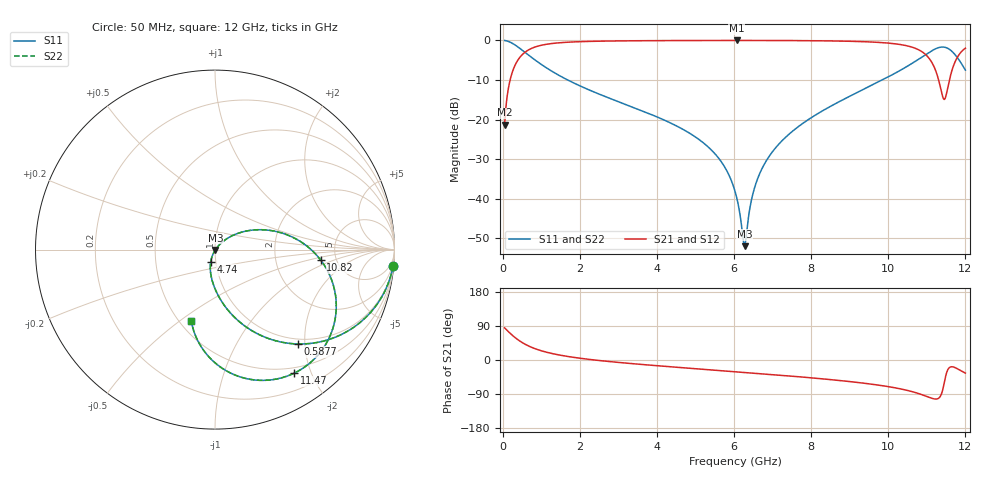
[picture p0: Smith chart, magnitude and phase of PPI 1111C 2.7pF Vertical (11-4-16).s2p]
# GHz S MA R 50
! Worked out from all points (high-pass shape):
!   1601 points, 50 MHz to 12 GHz, reference 50 ohm
!   highest |S21| = -0.02 dB at 6.07 GHz (marker M1); lowest = -21.3 dB at 50 MHz (marker M2)
!   |S21| within 3 dB of the highest: 575.9 MHz to 10.9 GHz (10.32 GHz wide, 180 % of centre); 11.88 GHz to end of sweep
!   lowest |S11| = -52.0 dB at 6.271 GHz (marker M3), VSWR 1.01, Z = 50.2 - j0.133 ohm
!   |S11| at or under -10 dB: 1.683 GHz to 9.847 GHz (8.163 GHz wide, 142 % of centre)
!   |S22| runs from -52.0 to 0.0 dB; largest |S21 - S12| = 0
!   S11 on the Smith chart (normalised r, x): 50 MHz: 1, -22; 587.8 MHz: 0.90, -1.86; 4.74 GHz: 0.94, -0.13; 10.82 GHz: 3.77, -0.68; 11.47 GHz: 0.42, -1.75; 12 GHz: 0.57, -0.55
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0.05  0.9963 -5.2  0.08604 84.8  0.08604 84.8  0.9963 -5.2
0.1545625  0.9661 -15.8  0.258 74.2  0.258 74.2  0.9661 -15.8
0.2516563  0.9169 -24.9  0.3988 65.1  0.3988 65.1  0.9169 -24.9
0.58775  0.7003 -48.7  0.7132 41.3  0.7132 41.3  0.7003 -48.7
1.140437  0.4477 -69.4  0.8932 20.5  0.8932 20.5  0.4477 -69.4
2.044156  0.2606 -85.6  0.9641 4.1  0.9641 4.1  0.2606 -85.6
4.038312  0.106 -104.4  0.9924 -15.4  0.9924 -15.4  0.106 -104.4
4.740375  0.0721 -109.4  0.9952 -20.9  0.9952 -20.9  0.0721 -109.4
5.569406  0.03391 -113.5  0.9969 -27.3  0.9969 -27.3  0.03391 -113.5
6.025  0.01241 -109.7  0.9972 -30.8  0.9972 -30.8  0.01241 -109.7
6.069813  0.01027 -107.5  0.9972 -31.1  0.9972 -31.1  0.01027 -107.5
6.271469  0.002511 -31.8  0.9971 -32.7  0.9971 -32.7  0.002511 -31.8
6.503  0.01222 43.1  0.9969 -34.5  0.9969 -34.5  0.01222 43.1
6.786812  0.02735 47.4  0.9965 -36.8  0.9965 -36.8  0.02735 47.4
7.272281  0.05562 46.0  0.9949 -40.7  0.9949 -40.7  0.05562 46.0
8.019156  0.1067 40.7  0.9899 -47.2  0.9899 -47.2  0.1067 40.7
10.01331  0.3484 17.1  0.9221 -70.5  0.9221 -70.5  0.3484 17.1
10.81994  0.5923 -5.7  0.7454 -89.7  0.7454 -89.7  0.5923 -5.7
11.20831  0.775 -30.4  0.4397 -102.9  0.4397 -102.9  0.775 -30.4
11.46972  0.8175 -57.4  0.1828 -51.2  0.1828 -51.2  0.8175 -57.4
11.73113  0.6602 -86.8  0.5339 -20.0  0.5339 -20.0  0.6602 -86.8
12  0.4204 -108.3  0.7958 -34.7  0.7958 -34.7  0.4204 -108.3
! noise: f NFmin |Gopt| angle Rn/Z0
0.05  0.0005808  0.9308  2.459  0.001866
1.372  0.003861  0.6835  9.133  0.00235
2.701  0.006159  0.6251  15.72  0.00302
4.031  0.008271  0.5968  22.25  0.00364
5.36  0.01044  0.5867  28.55  0.004351
6.682  0.01295  0.5939  34.54  0.005369
8.012  0.01665  0.626  40.36  0.007396
9.341  0.02492  0.7053  46.25  0.01412
10.67  0.06695  0.8679  52.55  0.08776
12  0.1153  0.915  58.58  0.2275
